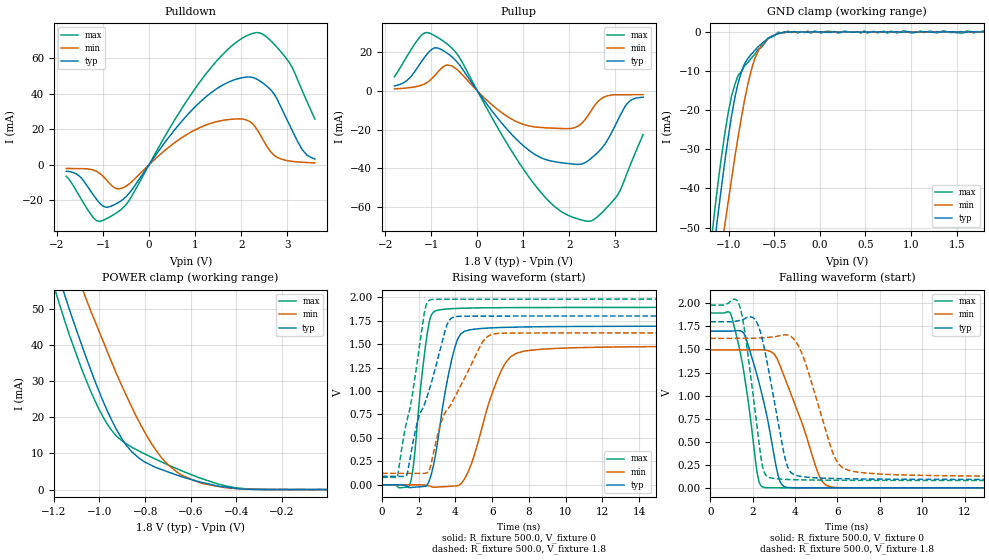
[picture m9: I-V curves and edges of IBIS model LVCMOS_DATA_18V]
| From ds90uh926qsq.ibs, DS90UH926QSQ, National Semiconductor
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[Model] LVCMOS_DATA_18V
Model_type 3-state
Enable Active-High
Vmeas = 0.9V
Cref = 0.0pF
Rref = 1.0e10
Vref = 0.0V
C_comp   2.75pF   2.32pF   3.18pF
[Voltage Range]   1.8V   1.62V   1.98V
[Temperature Range]   25.0   130.0   -40.0
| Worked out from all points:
|   slope of the pulldown table from 0 to 0.27 V, typ, clamps not added: 27.1 ohm
|   slope of the pullup table from 0 to 0.27 V, typ, clamps not added: 30.4 ohm
|   GND clamp passes 1 mA (typ) near -0.52 V on its own axis
|   POWER clamp passes 1 mA (typ) near -0.48 V on its own axis
|   rising waveform, R_fixture 500.0, V_fixture 0: 20-80 % time 891ps typ, 1.43ns min, 586ps max; typ from 0 V to 1.69 V
|   falling waveform, R_fixture 500.0, V_fixture 0: 20-80 % time 986ps typ, 1.37ns min, 718ps max; typ from 1.7 V to 0 V
|   rising waveform, R_fixture 500.0, V_fixture 1.8: 20-80 % time 1.52ns typ, 2.06ns min, 989ps max; typ from 0.09 V to 1.8 V
|   falling waveform, R_fixture 500.0, V_fixture 1.8: 20-80 % time 825ps typ, 1.18ns min, 626ps max; typ from 1.8 V to 0.09 V
[GND Clamp]
-1.8V     -191.5mA   -185.8mA   -202mA
-1.186V   -60.51mA   -74.09mA   -52.87mA
-1.148V   -52.87mA   -67.36mA   -44.82mA
-1.115V   -46.5mA    -61.8mA    -38.47mA
-1.038V   -32.65mA   -48.82mA   -25.52mA
-966.7mV  -21.44mA   -37.59mA   -16.38mA
-857.1mV  -10.05mA   -21.58mA   -10.08mA
-785.8mV  -6.698mA   -13.07mA   -7.761mA
-714.5mV  -4.764mA   -6.965mA   -5.776mA
-566.5mV  -1.583mA   -1.675mA   -1.668mA
-347.2mV  -97.28uA   -50.92uA   241.9uA
1.796V    44.94uA    0A         278.7uA
[POWER Clamp]
-1.8V     189.4mA    185.2mA    199.2mA
-1.186V   60.43mA    74.18mA    53.54mA
-1.148V   52.96mA    67.56mA    45.82mA
-1.06V    36.85mA    53.03mA    30.51mA
-966.7mV  21.93mA    38.4mA     18.2mA
-879mV    12mA       25.6mA     12.52mA
-769.3mV  6.604mA    12.45mA    8.881mA
-714.5mV  5.229mA    7.863mA    7.264mA
-659.7mV  3.981mA    4.813mA    5.735mA
-550.1mV  1.973mA    1.699mA    2.998mA
-402mV    324.8uA    274.3uA    472.1uA
-1.827mV  -2.763uA   -12.28uA   -3.061uA
[Pullup]
-1.8V     2.538mA    1.037mA    7.355mA
-1.148V   17.33mA    3.544mA    29.96mA
-714.5mV  20.36mA    12.9mA     25.27mA
-385.6mV  13.35mA    9.771mA    17.08mA
431.3mV   -13.8mA    -9.46mA    -18.61mA
1.034V    -29.1mA    -17.59mA   -41.6mA
1.687V    -36.62mA   -19.31mA   -59.93mA
2.345V    -37.01mA   -14.68mA   -67.18mA
2.668V    -30.55mA   -4.513mA   -63.79mA
3.052V    -15.17mA   -1.997mA   -53.63mA
3.326V    -4.849mA   -1.98mA    -38.08mA
3.6V      -3.327mA   -1.965mA   -22.59mA
[Pulldown]
-1.8V     -3.706mA   -2.144mA   -6.494mA
-1.477V   -7.386mA   -2.221mA   -19.29mA
-1.148V   -19.3mA    -3.654mA   -31.36mA
-928.3mV  -23.95mA   -8.523mA   -30.41mA
-659.7mV  -21.18mA   -13.63mA   -26.23mA
1.144V    36.07mA    21.32mA    47.95mA
1.961V    48.52mA    25.76mA    70.05mA
2.29V     48.71mA    21.73mA    74.06mA
2.668V    41.3mA     6.532mA    69.02mA
3.052V    22.21mA    2.071mA    57.14mA
3.326V    8.437mA    1.359mA    41.62mA
3.6V      3.223mA    999uA      25.67mA
[Rising Waveform]
R_fixture=500.0
V_fixture=0
V_fixture_min=0
V_fixture_max=0
0s        22.28nV    566nV      3.79nV
1.55ns    -29.42mV   232.4nV    25.47mV
2.5ns     13.24mV    -7.986mV   1.662V
3.05ns    489.1mV    -23.95mV   1.863V
3.7ns     1.251V     -15.91mV   1.877V
4.3ns     1.611V     12.3mV     1.882V
4.9ns     1.656V     242.3mV    1.886V
6.45ns    1.678V     1.198V     1.889V
7.75ns    1.684V     1.426V     1.89V
49.98ns   1.694V     1.484V     1.893V
[Falling Waveform]
R_fixture=500.0
V_fixture=0
V_fixture_min=0
V_fixture_max=0
0s        1.699V     1.495V     1.895V
1ns       1.699V     1.495V     1.861V
1.6ns     1.668V     1.495V     1.228V
2.2ns     1.225V     1.496V     178.8mV
2.55ns    904.3mV    1.494V     4.087mV
3.15ns    183.2mV    1.401V     698uV
3.35ns    43.9mV     1.29V      575.1uV
5.1ns     494.1uV    150mV      213.1uV
5.75ns    355.2uV    7.966mV    158.8uV
49.98ns   4.738uV    12.73uV    3.918uV
[Rising Waveform]
R_fixture=500.0
V_fixture=1.8
V_fixture_min=1.62
V_fixture_max=1.98
0s        90.38mV    122.1mV    79.85mV
850ps     90.38mV    122.1mV    98.02mV
1.35ns    105.8mV    122.1mV    682.3mV
2.3ns     852mV      121.4mV    1.831V
2.65ns    1.064V     205.6mV    1.974V
3.25ns    1.51V      683.7mV    1.978V
3.7ns     1.762V     839.9mV    1.979V
5.45ns    1.799V     1.514V     1.98V
6.2ns     1.799V     1.612V     1.98V
49.98ns   1.8V       1.62V      1.98V
[Falling Waveform]
R_fixture=500.0
V_fixture=1.8
V_fixture_min=1.62
V_fixture_max=1.98
0s        1.8V       1.62V      1.98V
1.35ns    1.812V     1.62V      1.991V
2.05ns    1.839V     1.62V      951.6mV
2.45ns    1.613V     1.626V     249mV
2.9ns     1.088V     1.633V     105.5mV
3.8ns     166.1mV    1.641V     89.32mV
4.4ns     119.9mV    1.41V      86.05mV
5.9ns     101mV      316.3mV    82.45mV
7ns       96.63mV    169.2mV    81.41mV
49.98ns   90.38mV    122.1mV    79.85mV
[Ramp]
R_load = 500.0
dV/dt_r   1.016291E0/9E-10   8.905759E-1/1.45E-9   1.135649E0/5.5E-10
dV/dt_f   1.02577E0/8.5E-10   8.987497E-1/1.2E-9   1.14009E0/6.5E-10
